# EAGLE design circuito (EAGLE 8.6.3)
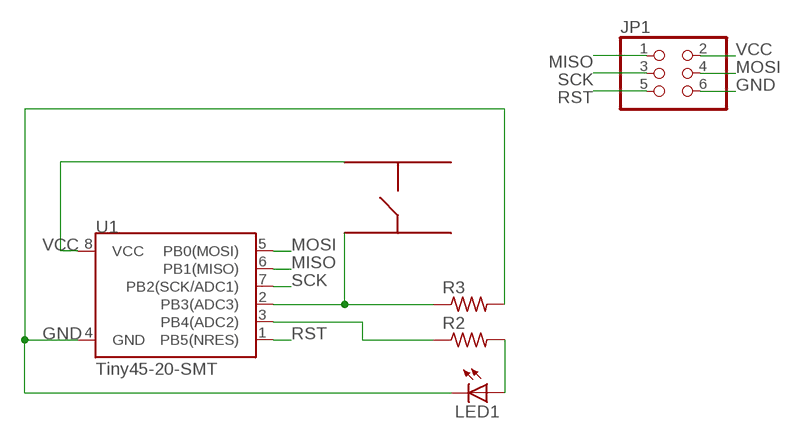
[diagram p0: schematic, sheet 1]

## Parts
JP1  PINHD-2X3  [2X03]
LED1  LEDCHIPLED_1206  [CHIPLED_1206]
R2  R-US_R1206  [R1206]
R3  R-US_R1206  [R1206]
S1  TACTSWITCH  [TACT]
U1  Tiny45-20-SMT  ATTINY45TINY45-20-SMT  [SO08-EIAJ]

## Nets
GND: JP1.6 LED1.C R3.2 U1.4(GND)
MISO: JP1.1 U1.6(PB1(MISO))
MOSI: JP1.4 U1.5(PB0(MOSI))
N$1: R2.1 U1.3(PB4(ADC2))
N$3: LED1.A R2.2
N$8: R3.1 S1.3 U1.2(PB3(ADC3))
RST: JP1.5 U1.1(PB5(NRES))
SCK: JP1.3 U1.7(PB2(SCK/ADC1))
VCC: JP1.2 S1.1 U1.8(VCC)
Unconnected: S1.2 S1.4

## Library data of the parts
JP1 = pinhead:PINHD-2X3: PIN HEADER
LED1 = led:LED: LED
R2 R3 = resistor:R-US_: RESISTOR, American symbol
S1 = oliver:TACTSWITCH
U1 = SparkFun-DigitalIC:ATTINY45: Atmel 8-pin 2/4/8kB flash uC; PROD_ID: IC-08922

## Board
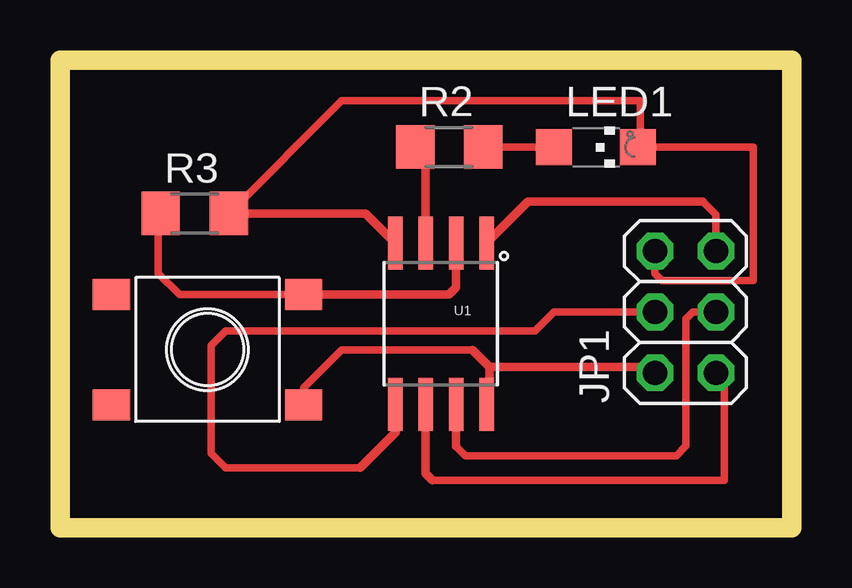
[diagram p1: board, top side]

Size 30.5 x 19.5 mm. Coordinates in mm from the lower left corner, seen from the top.
Outline: 0,0 30.5,0 30.5,19.5 0,19.5 0,0
Copper layers (1*16): Top 0.035mm / dielectric 1.5mm / Bottom 0.035mm
Design rules "default *": minimum track width 12mil, minimum drill 24mil, track to track 10mil, track to pad 10mil, pad to pad 10mil, via to via 10mil, smd to smd 8mil, copper to edge 40mil, drill to drill 8mil, minimum pad ring 10mil, minimum via ring 8mil, stop-mask expansion 4mil, vias tented up to drill 0mil, thermal gap 10mil

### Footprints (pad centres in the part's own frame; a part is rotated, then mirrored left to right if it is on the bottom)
2X03 = drill 1.016 octagon: 1 -2.54,-1.27; 2 -2.54,1.27; 3 0,-1.27; 4 0,1.27; 5 2.54,-1.27; 6 2.54,1.27
CHIPLED_1206 = smd 1.5 x 1.5: A 0,-1.75; C 0,1.75
R1206 = smd 1.6 x 1.803: 1 -1.422,0; 2 1.422,0
TACT = smd 1.55 x 1.3: 1 -4,2.3; 2 4,2.3; 3 -4,-2.3; 4 4,-2.3
SO08-EIAJ = smd 0.61 x 2.21: 1 -1.905,-3.378; 2 -0.635,-3.378; 3 0.635,-3.378; 4 1.905,-3.378; 5 1.905,3.353; 6 0.635,3.353; 7 -0.635,3.353; 8 -1.905,3.353

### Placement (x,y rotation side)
JP1  26.08,8.99 90 top
LED1  22.35,15.86 270 top
R2  16.23,15.87 0 top
R3  5.62,13.1 0 top
S1  6.15,7.42 180 top
U1  15.88,8.49 180 top

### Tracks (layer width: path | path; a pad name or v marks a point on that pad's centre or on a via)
GND
  Top 0.305: R3.2 11.74,17.8 24.2,17.8 24.2,15.96 LED1.C 28.9,15.86 28.9,10.3 25.1,10.3 24.81,10.59 JP1.6
  Top 0.356: U1.4 12.74,13.1 R3.2
MISO
  Top 0.305: 15.53,1.97 27.7,1.97 27.7,6.1 JP1.1
  Top 0.356: U1.6 15.24,2.25 15.53,1.97
MOSI
  Top 0.305: JP1.4 20.59,8.99 19.8,8.2 6.9,8.2 6.3,7.6 6.3,3.1 6.9,2.5 12.5,2.5 | 14,4 13.97,4.03 U1.5
  Top 0.356: 12.5,2.5 14,4
N$1
  Top 0.305: 15.24,15.43 R2.1
  Top 0.356: U1.3 15.24,15.43
N$3
  Top 0.305: LED1.A 17.66,15.86 R2.2
N$8
  Top 0.305: R3.1 4.1,13 4.1,10.6 4.98,9.72 S1.3
  Top 0.356: U1.2 16.52,10.02 16.22,9.72 S1.3
RST
  Top 0.305: JP1.5 27.35,13.05 26.8,13.6
  Top 0.356: U1.1 19.52,13.6 26.8,13.6
SCK
  Top 0.305: JP1.3 26.39,8.99 26.1,8.7 26.1,3.4 25.7,3 16.9,3 16.52,3.38
  Top 0.356: 16.52,3.38 U1.7
VCC
  Top 0.305: 17.2,7.4 11.73,7.4 10.15,5.82 S1.1 | U1.8 17.9,5.25 | 24.56,6.7 JP1.2
  Top 0.356: 17.9,6.7 17.2,7.4 | 17.9,5.25 17.9,6.7 | 17.9,6.7 24.56,6.7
